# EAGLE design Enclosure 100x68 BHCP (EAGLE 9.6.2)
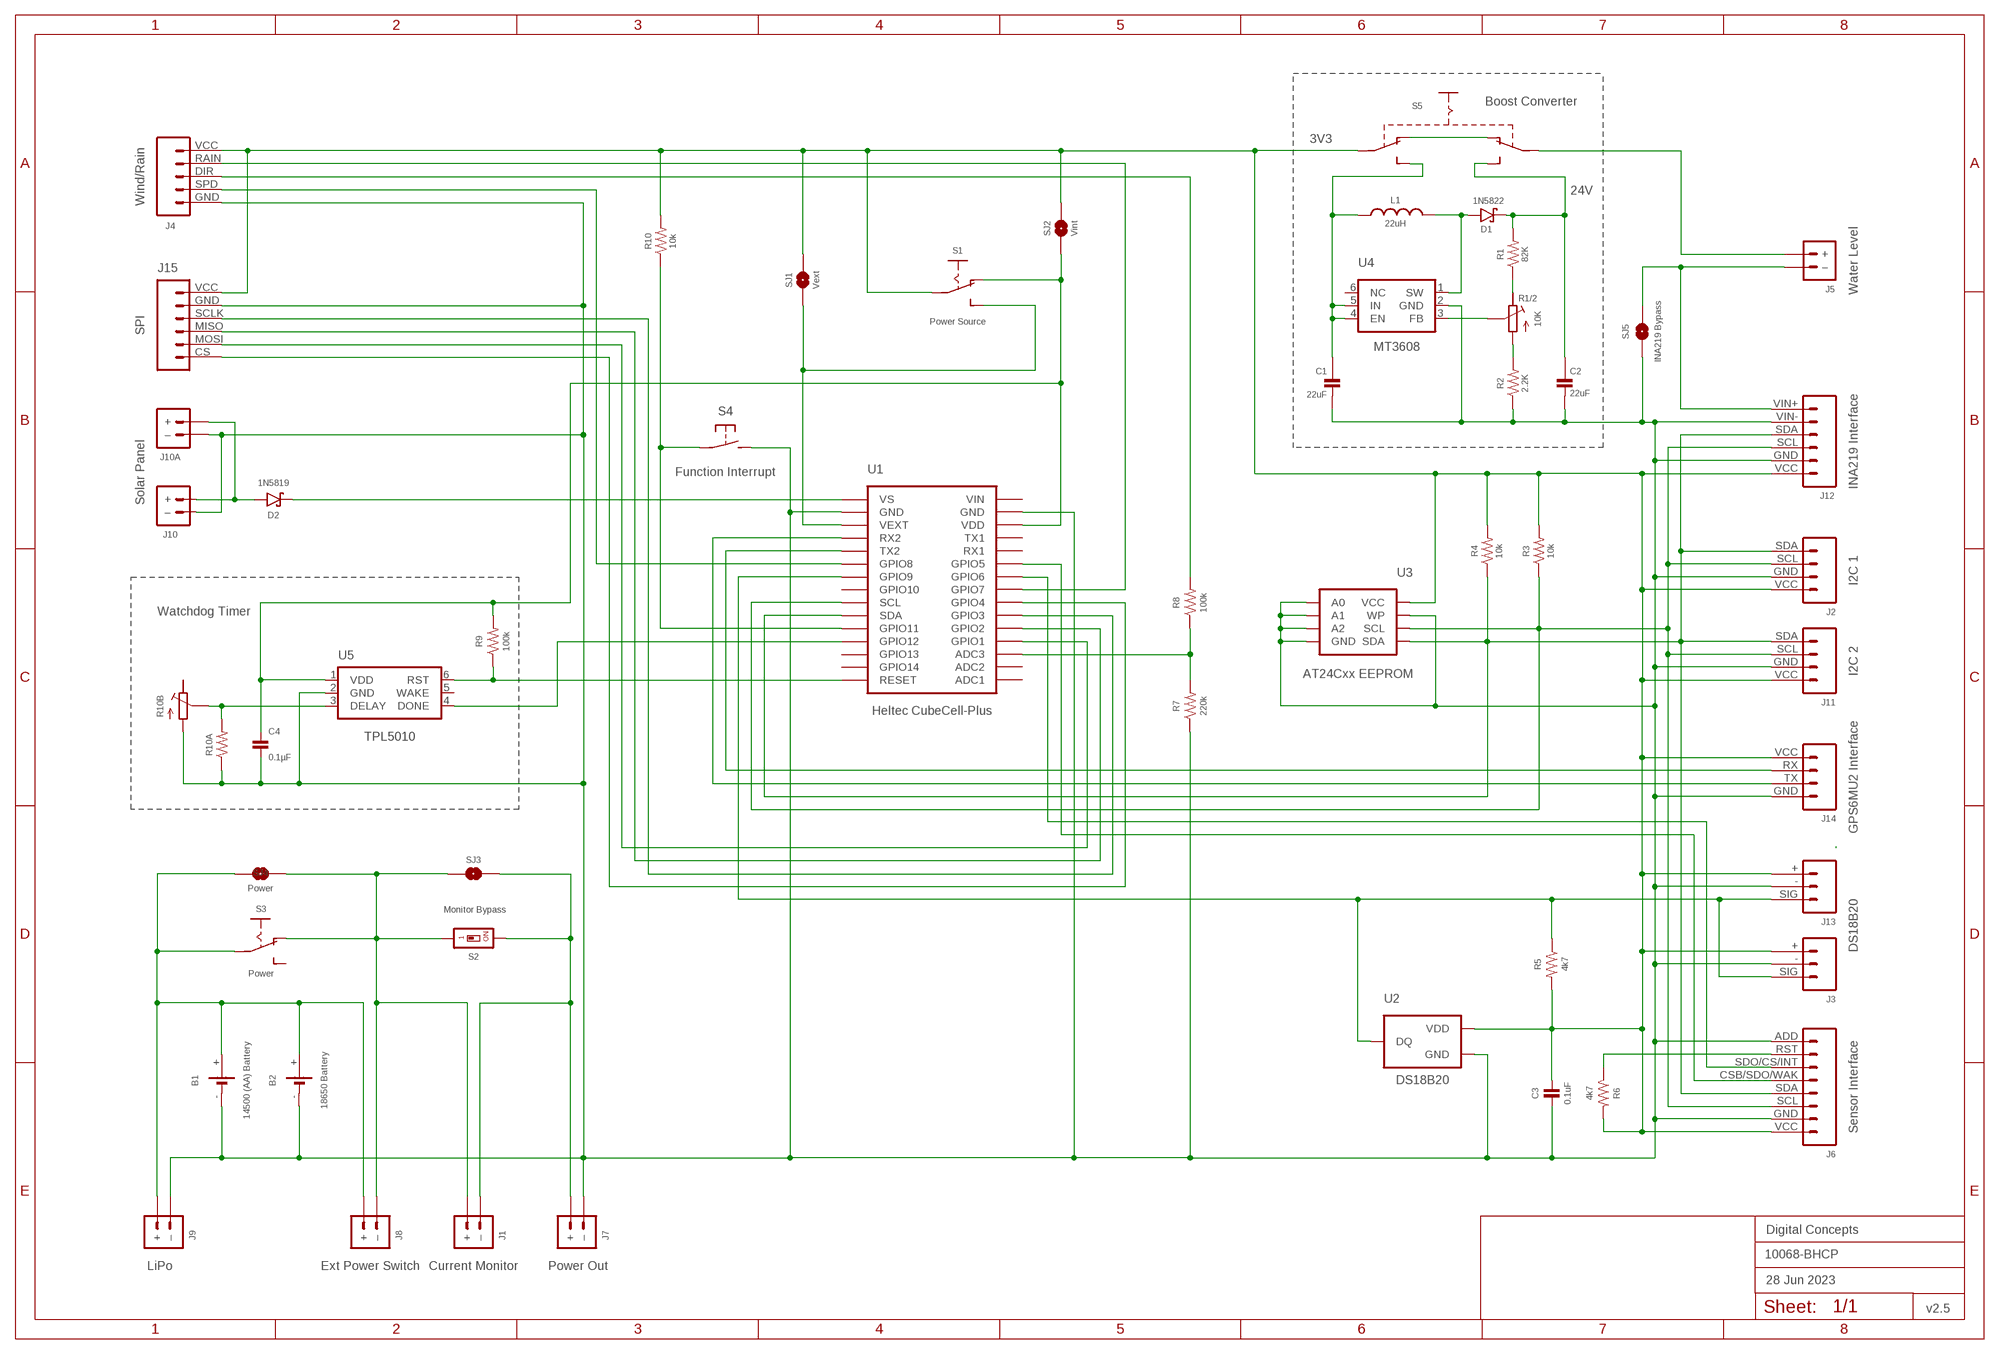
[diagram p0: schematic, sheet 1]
FRAME2 (A3L-LOC): DATE: 28 Jun 2023; OWNER: Digital Concepts; TITLE: 10068-BHCP; VERSION: v2.5

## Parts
B1  14500 (AA) Battery  BATTERY-HOLDER-14500(AA)  [BATTERY-14500]
B2  18650 Battery  BATTERY-HOLDER-18650  [BATTERY-18650]
C1  22uF  CAPACITOR-1206  [C1206]
C2  22uF  CAPACITOR-1206  [C1206]
C3  0.1uF  CAPACITOR-0805  [C0805]
C4  0.1µF  CAPACITOR-0805  [C0805]
D1  1N5822  DIODE-SCHOTTKY-1N5822  [DIODE_SMB]
D2  1N5819  1N5819-SOD-123  [SOD-123]
J1  Current Monitor  JST-PH2.0-2-HORIZONTALJST-PTH-2  [JST-PH2.0-2-HORIZONTAL]
J2  I2C 1  JST-PH2.0-4-VERTICAL-I2C  [JST-PH2.0-4-VERTICAL-I2C]
J3  DS18B20  JST-PH2.0-3-VERTICAL-DS18B20  [JST-PH2.0-3-VERTICAL-SIG]
J4  Wind/Rain  JST-PH2.0-5-DUAL-WEATHER  [JST-PH2.0-5-DUAL-WEATHER]
J5  Water Level  JST-PH2.0-2-DUAL-POWERJST-PTH-2  [JST-PH2.0-2-DUAL-POWER]
J6  Sensor Interface  HEADER-1X8-SENSOR  [CONN_08-SENSOR]
J7  Power Out  JST-GH1.25-2-HORIZONTAL-POWER  [JST-GH1.25-2-HORIZONTAL]
J8  Ext Power Switch  JST-PH2.0-2-DUAL-POWERJST-PTH-2  [JST-PH2.0-2-DUAL-POWER]
J9  LiPo  JST-PH2.0-2-HORIZONTAL-POWERJST-PTH-2  [JST-PH2.0-2-HORIZONTAL-POWER]
J10  Solar Panel  JST-PH2.0-2-VERTICAL  [JST-PH2.0-2-VERTICAL=POWER]
J10A  JST-PH2.0-2-HORIZONTAL-POWERJST-PTH-2  [JST-PH2.0-2-HORIZONTAL-POWER]
J11  I2C 2  JST-PH2.0-I2C-MALE-HORIZONTAL  [JST-PH2.0-4-HORIZONTAL]
J12  INA219 Interface  INA219-I2C-MODULE  [CONN_06-INA219]
J13  JST-PH2.0-3-HORIZONTAL-DS18B20  [JST-PH2.0-DS18B20-HORIZONTAL]
J14  GPS6MU2 Interface  HEADER-1X4-GPS  [CONN_04-GPS]
J15  SPI  JST-PH2.0-6-HORIZONTAL-SPI  [JST-PH2.0-6-HORIZONTAL-SPI]
L1  22uH  INDUCTOR-CDRH104R/6D28L5038P  [CDRH104R+6D28]
R1  82K  RESISTORR0805  [R0805]
R1/2  10K  RESISTOR-TRIMM-BAOTER-HORIZONTAL  [RTRIM64P]
R2  2.2K  RESISTORR0805  [R0805]
R3  10k  RESISTORR0805  [R0805]
R4  10k  RESISTORR0805  [R0805]
R5  4k7  RESISTORR0805  [R0805]
R6  4k7  RESISTORR0805  [R0805]
R7  220k  RESISTORR0805  [R0805]
R8  100k  RESISTORR0805  [R0805]
R9  100k  RESISTORR0805  [R0805]
R10  10k  RESISTORR0805  [R0805]
R10A  RESISTORR0805  [R0805]
R10B  RESISTOR-TRIMM-33  [RTRIM3*3]
S1  Power Source  SWITCH-SLIDE-SPDT-SMT  [SWITCH-SPDT-SMT]
S2  Monitor Bypass  SWITCH-DIP-SWS001  [SMD-001]
S3  Power  SWITCH-SLIDE-SPDT-PTH  [SWITCH-SPDT-PTH]
S4  Function Interrupt  SWITCH-MOMENTARY-2-PIN  [SWITCH-2-PAD]
S5  SWITCH-SLIDE-DPDT-PTH-S  [SWITCH-DPDT-PTH]
SJ1  Vext  SJ  [SJ]
SJ2  Vint  SJ-V-12  [SJ-VIA-12]
SJ3  Monitor  SJ  [SJ]
SJ4  Power  SJ  [SJ]
SJ5  INA219 Bypass  SJ  [SJ]
U1  Heltec CubeCell-Plus  HELTEC-CUBECELL-PLUS-X  [HELTEC-CUBECELL=PLUS-X]
U2  DS18B20  THERMOMETER-DS18B20  [TO-92]
U3  AT24Cxx EEPROM  AT24CXX-EEPROM  [SOP-8]
U4  MT3608  [SOT-23-6]
U5  TPL5010  TPL5010DDCR  [SOT-23-6]

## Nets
GND: B1.- B2.- C1.2 C2.2 C3.2 C4.2 J2.GND J3.- J4.GND J6.ADD J6.GND J7.-(–) J9.-(–) J10.-(–) J10A.-(–) J11.GND J12.GND J12.VIN- J13.- J14.GND J15.GND R2.1 R7.1 R10A.1 R10B.1(A) S4.P$2(S) SJ5.1 U1.GND@14(GND) U1.GND@17(GND) U2.1(GND) U3.P$1(A0) U3.P$2(A1) U3.P$3(A2) U3.P$4(GND) U3.P$7(WP) U4.2(GND) U5.2(GND)
N$1: D2.A J10.+ J10A.+
N$2: R7.2 R8.1 U1.ADC3
N$3: J1.2(–) J7.+ S2.2 SJ3.1
N$4: B1.+ B2.+ J8.+ J9.+ S3.2(P) SJ4.2
N$5: D2.C U1.VS
N$6: D1.A L1.1 U4.1(SW)
N$7: J4.DIR R8.2
N$8: J2.SCL J6.SCL J11.SCL J12.SCL R3.1 U1.SCL U3.P$6(SCL)
N$9: J6.RST R6.1
N$10: J6.CSB/SDO/WAK U1.GPIO5
N$11: J2.SDA J6.SDA J11.SDA J12.SDA R4.1 U1.SDA U3.P$5(SDA)
N$12: J4.SPD U1.GPIO8
N$13: S1.3(S) SJ1.1 U1.VEXT
N$14: J14.RX U1.TX2
N$15: J5.-(–) J12.VIN+ SJ5.2
N$16: J14.TX U1.RX2
N$18: R10A.2 R10B.2(S) U5.3(DELAY)
N$19: J6.SDO/CS/INT U1.GPIO6
N$20: J5.+ S5.P$2(P1)
N$21: J1.1(+) J8.-(–) S2.1 S3.1(O) SJ3.2 SJ4.1
N$22: R1/2.2(S) U4.3(FB)
N$23: R1/2.1(A) R2.2
N$24: J3.SIG J13.SIG R5.1 U1.GPIO9 U2.2(DQ)
N$25: C1.1 L1.2 S5.P$6(S2) U4.4(EN) U4.5(IN)
N$26: S5.P$1(O1) S5.P$4(O2)
N$27: R10.1 S4.P$1(P) U1.GPIO11
N$28: C2.1 D1.C R1.2 S5.P$3(S1)
N$29: J15.MOSI U1.GPIO1
N$30: J15.MISO U1.GPIO2
N$32: J4.RAIN U1.GPIO7
N$34: R9.1 U1.RST(RESET) U5.6(RST)
N$35: J15.SCLK U1.GPIO3
N$36: J15.CS U1.GPIO4
N$37: U1.GPIO12 U5.4(DONE)
N$38: R1.1 R1/2.3(E)
N$39: C4.1 R9.2 S1.1(O) SJ2.1 SJ2.1@V U1.VDD U5.1(VDD)
VEXT: C3.1 J2.VCC J3.+ J4.VCC J6.VCC J11.VCC J12.VCC J13.+ J14.VCC J15.VCC R3.2 R4.2 R5.2 R6.2 R10.2 S1.2(P) S5.P$5(P2) SJ1.2 SJ2.2 SJ2.2@V U2.3(VDD) U3.P$8(VCC)
Unconnected: R10B.3(E) S3.3(S) U1.ADC1 U1.ADC2 U1.GPIO10 U1.GPIO13 U1.GPIO14 U1.RX1 U1.TX1 U4.6(NC) U5.5(WAKE)

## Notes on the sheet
- Boost Converter
- 3V3
- 24V
- Watchdog Timer

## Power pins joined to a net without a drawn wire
VIN: U1.VIN

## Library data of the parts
B1 = digitalconcepts:BATTERY-HOLDER-14500(AA): 14500 (AA) battery holder
B2 = digitalconcepts:BATTERY-HOLDER-18650: 18650 Battery Holder
C1 C2 = digitalconcepts:CAPACITOR-1206: 1206 Capacitor
C3 C4 = digitalconcepts:CAPACITOR-0805: 0805 Capacitor
D1 = digitalconcepts:DIODE-SCHOTTKY-1N5822: 1N5822 Schottky Diode SMB
D2 = digitalconcepts:1N5819-SOD-123: 1N5819 Schottky Diode SOD-123
J1 = digitalconcepts:JST-PH2.0-2-HORIZONTAL: PH2.0 2P Right Angle PCB Connector; PROD_ID: CONN-09863; SKU: PRT-09914
J2 = digitalconcepts:JST-PH2.0-4-VERTICAL-I2C: PH2.0 4P I2C Vertical Connector
J3 = digitalconcepts:JST-PH2.0-3-VERTICAL-DS18B20: DS18B20 PH2.0 Vertical PCB Connector
J4 = digitalconcepts:JST-PH2.0-5-DUAL-WEATHER: PH2.0 5P Dual Connector
J5 J8 = digitalconcepts:JST-PH2.0-2-DUAL-POWER: JST PH2.0 2P PTH Dual-Side Connector (Power); PROD_ID: CONN-09863; SKU: PRT-09914
J6 = digitalconcepts:HEADER-1X8-SENSOR: IoT Sensors 1x8 Pin Header for 'Sandwich' IoT Sensors
J7 = digitalconcepts:JST-GH1.25-2-HORIZONTAL-POWER: JST GH1.25 2P PTH Connector (Power)
J9 J10A = digitalconcepts:JST-PH2.0-2-HORIZONTAL-POWER: PH2.0 2P Right Angle PCB Connector; PROD_ID: CONN-09863; SKU: PRT-09914
J10 = digitalconcepts:JST-PH2.0-2-VERTICAL: PH2.0 2P PCB Connector
J11 = digitalconcepts:JST-PH2.0-I2C-MALE-HORIZONTAL: PH2.0 4P (I2C) Right Angle PCB Connector
J12 = digitalconcepts:INA219-I2C-MODULE: INA219 I2C Module
J13 = digitalconcepts:JST-PH2.0-3-HORIZONTAL-DS18B20: DS18B20 PH2.0 Right Angle PCB Connector
J14 = digitalconcepts:HEADER-1X4-GPS: NEO GPS 4-Pin Header
J15 = digitalconcepts:JST-PH2.0-6-HORIZONTAL-SPI: PH2.0 6P Horizontal Connector—SPI
L1 = digitalconcepts:INDUCTOR-CDRH104R/6D28: Inductor; SPICEPREFIX: L
R1-R10 R10A = digitalconcepts:RESISTOR: Resistor; SPICEPREFIX: R
R1/2 = digitalconcepts:RESISTOR-TRIMM-BAOTER-HORIZONTAL: Trimm Resistor - Horizontal BAOTER
R10B = digitalconcepts:RESISTOR-TRIMM-3*3: Trimm Resistor - 3*3 SMD
S1 = digitalconcepts:SWITCH-SLIDE-SPDT-SMT: Mini Sliding Switch SPDT SMT
S2 = digitalconcepts:SWITCH-DIP-SWS001: SMD Dip Switch 1 pol.
S3 = digitalconcepts:SWITCH-SLIDE-SPDT-PTH: Mini Sliding Switch SPDT PTH
S4 = digitalconcepts:SWITCH-MOMENTARY-2-PIN: 2 Pin Momentary Switch
S5 = digitalconcepts:SWITCH-SLIDE-DPDT-PTH-S: Switch DPDT PTH-S
SJ1 SJ3-SJ5 = digitalconcepts:SJ: Solder Jumper
SJ2 = digitalconcepts:SJ-V-12: Solder Jumper with Pad Vias
U1 = digitalconcepts:HELTEC-CUBECELL-PLUS-X: Heltec CubeCell Dev-Board Plus Excluding internal pins
U2 = digitalconcepts:THERMOMETER-DS18B20: Digital Thermometer -55C-125C TO92-3; AVAILABILITY: Bad; DESCRIPTION: Temperature Sensor Digital, Local -55°C ~ 125°C 12 b 8-uMAX; MF: Maxim Integrated; MP: DS18B20; PACKAGE: TO-92 Maxim Integrated; PRICE: None
U3 = digitalconcepts:AT24CXX-EEPROM: AT24Cxx EEPROM SOP-8
U4 = digitalconcepts:MT3608: MT3608 DC-DC Step-Up Voltage Converter
U5 = digitalconcepts:TPL5010DDCR: TPL5010 Nano-Power System Timer with Watchdog

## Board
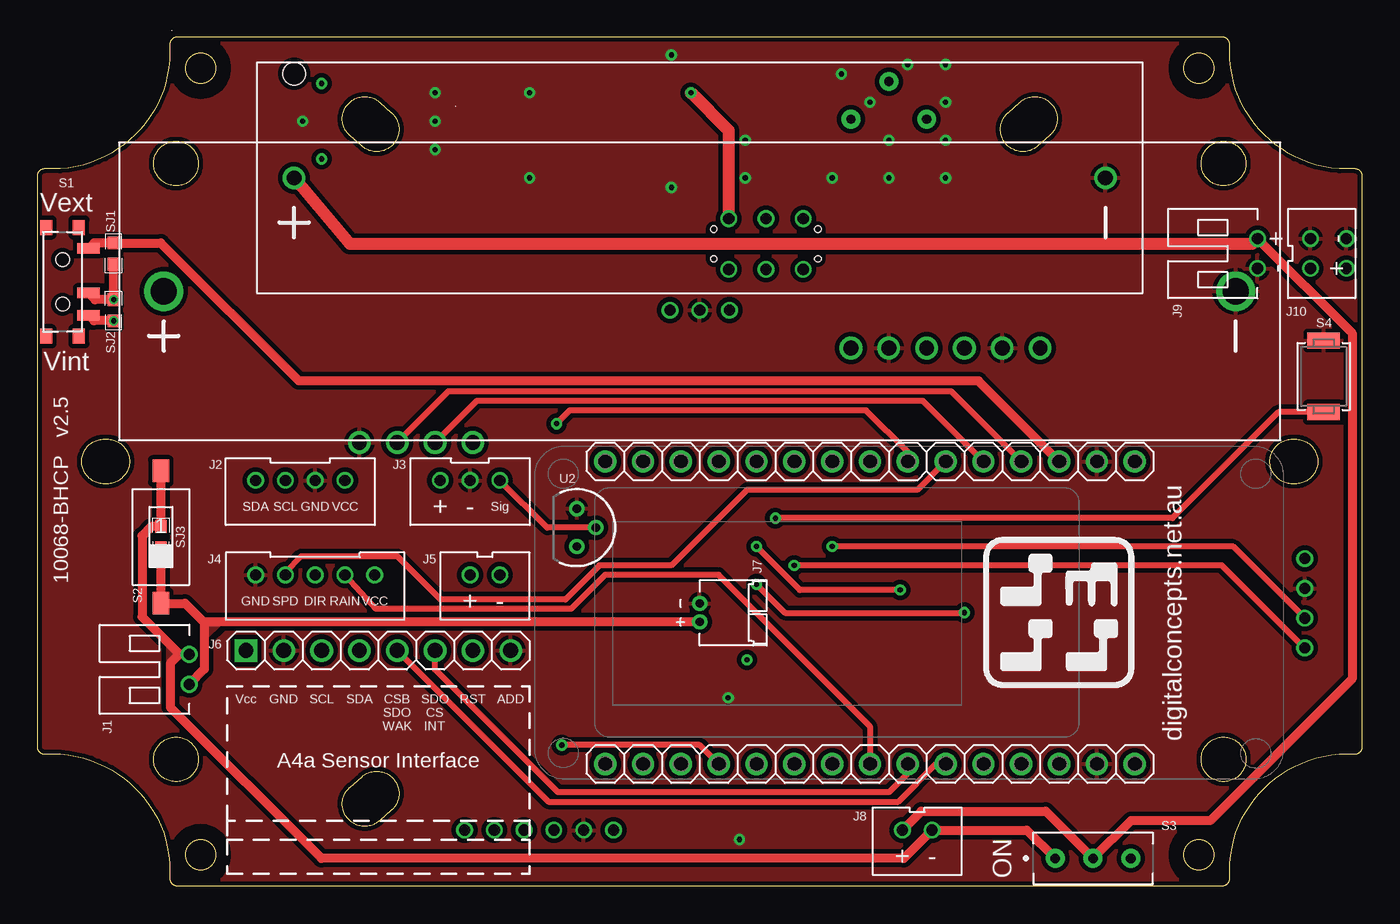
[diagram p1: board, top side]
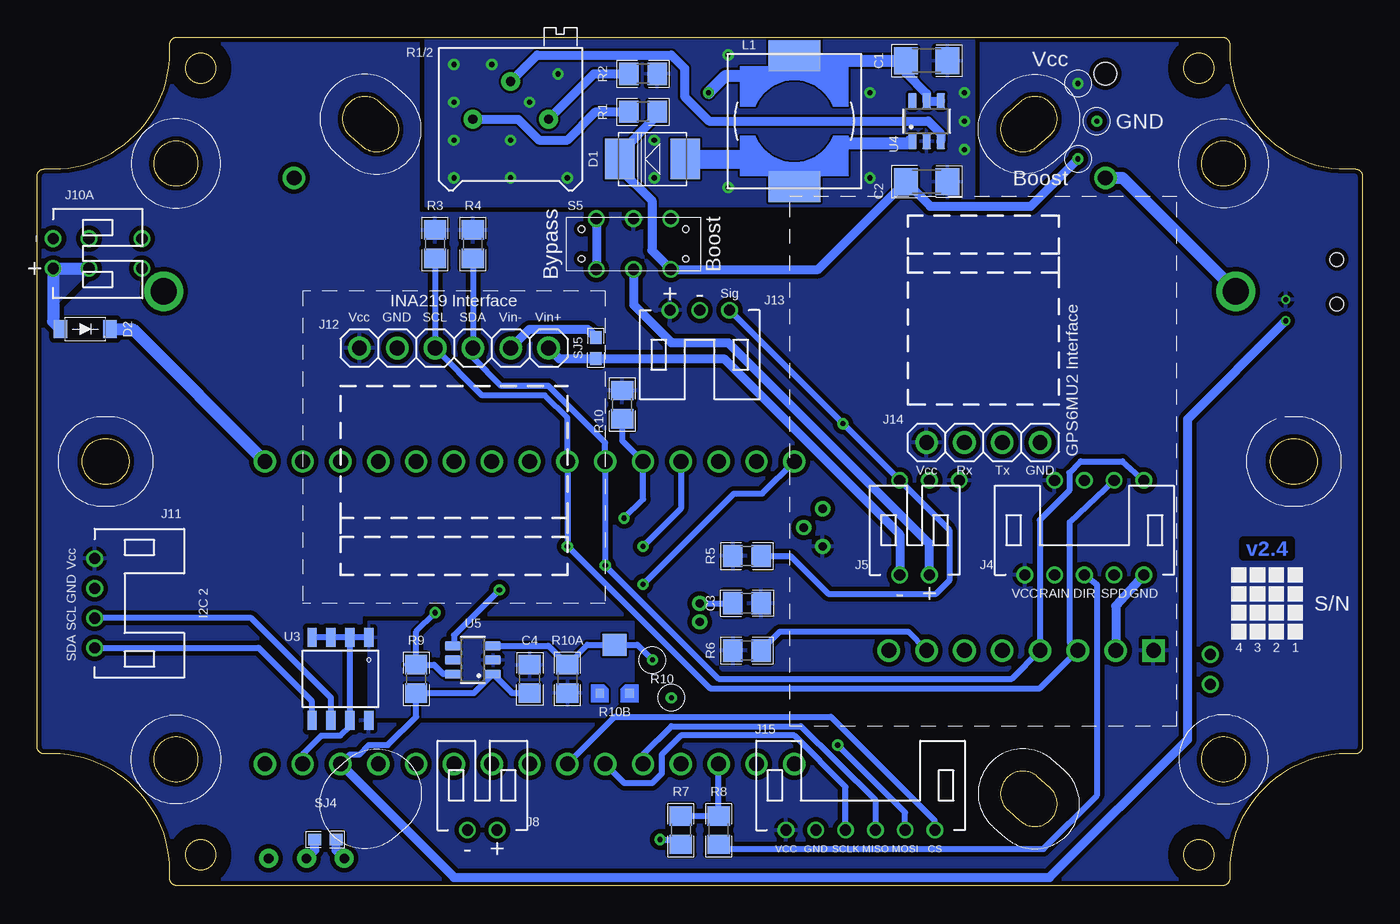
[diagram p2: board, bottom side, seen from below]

Size 89 x 57 mm. Coordinates in mm from the lower left corner, seen from the top.
Outline: 1134 segments
Outline: circle at 10.97,2.08 radius 1.02
Outline: circle at 10.97,54.92 radius 1.02
Outline: circle at 78.03,54.92 radius 1.02
Outline: circle at 78.03,2.08 radius 1.02
Copper layers (1*16): Top 0.035mm / dielectric 1.5mm / Bottom 0.035mm
Design rules "default *": minimum track width 6mil, minimum drill 0.35mm, track to track 6mil, track to pad 6mil, pad to pad 6mil, via to via 6mil, smd to smd 6mil, copper to edge 6mil, drill to drill 6mil, minimum pad ring 1mil, minimum via ring 8mil, stop-mask expansion 4mil, vias tented up to drill 0mil, thermal gap 10mil

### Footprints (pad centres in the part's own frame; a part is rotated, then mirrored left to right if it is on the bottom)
BATTERY-14500 = drill 1: + -27.25,0; - 27.25,0 | hole 1.524: -27.25,7
BATTERY-18650 = drill 1.75: + -36,0; - 36,0
C1206 = smd 1.6 x 1.8: 1 -1.4,0; 2 1.4,0
C0805 = smd 1.3 x 1.5: 1 -0.95,0; 2 0.95,0
DIODE_SMB = smd 2 x 2.7: A 2.2,0; C -2.2,0
SOD-123 = smd 0.91 x 1.22: A -1.65,0; C 1.65,0
JST-PH2.0-2-HORIZONTAL = drill 0.75: 1 1,0; 2 -1,0
JST-PH2.0-4-VERTICAL-I2C = drill 0.75: GND 1,0; SCL -1,0; SDA -3,0; VCC 3,0
JST-PH2.0-3-VERTICAL-SIG = drill 0.75: + -2,0; - 0,0; SIG 2,0
JST-PH2.0-5-DUAL-WEATHER = drill 0.75: DIR 0,0; GND 4,0; RAIN -2,0; SPD 2,0; VCC -4,0
JST-PH2.0-2-DUAL-POWER = drill 0.75: + 1,0; - -1,0
CONN_08-SENSOR = drill 1 pad 1.524: ADD 17.78,0; CSB/SDO/WAK 10.16,0; GND 2.54,0; RST 15.24,0; SCL 5.08,0; SDA 7.62,0; SDO/CS/INT 12.7,0 | drill 1 pad 1.524 square: VCC 0,0
JST-GH1.25-2-HORIZONTAL = drill 0.55 pad 1.016: + -0.625,0; - 0.625,0
JST-PH2.0-2-HORIZONTAL-POWER = drill 0.75: + 1,0; - -1,0
JST-PH2.0-2-VERTICAL=POWER = drill 0.75: + -1,0; - 1,0
JST-PH2.0-4-HORIZONTAL = drill 0.75: GND -1,0; SCL 1,0; SDA 3,0; VCC -3,0
CONN_06-INA219 = drill 1 pad 1.524: GND 2.54,0; SCL 5.08,0; SDA 7.62,0; VCC 0,0; VIN+ 12.7,0; VIN- 10.16,0
JST-PH2.0-DS18B20-HORIZONTAL = drill 0.75: + 2,0; - 0,0; SIG -2,0
CONN_04-GPS = drill 1 pad 1.524: GND 0,0; RX 5.08,0; TX 2.54,0; VCC 7.62,0
JST-PH2.0-6-HORIZONTAL-SPI = drill 0.75: CS 5,0; GND -3,0; MISO 1,0; MOSI 3,0; SCLK -1,0; VCC -5,0
CDRH104R+6D28 = smd 2.1 x 3.5: 1 -4.4,0; 2 4.4,0
R0805 = smd 1.3 x 1.5: 1 -0.95,0; 2 0.95,0
RTRIM64P = drill 0.61 pad 1.27: 1 0,-2.54; 2 2.54,0; 3 0,2.54
RTRIM3*3 = smd 0.6 x 0.6: 1 -1,-1.6; 3 1,-1.6 | smd 1.6 x 1.5: 2 0,1.65
SWITCH-SPDT-SMT = smd 0.7 x 1.5: 1 2.25,1.75; 2 0.75,1.75; 3 -2.25,1.75 | smd 1 x 0.8: GND@1 3.65,-1.1; GND@2 3.65,1.1; GND@3 -3.65,1.1; GND@4 -3.65,-1.1 | hole 0.9: -1.5,0; 1.5,0
SMD-001 = smd 1.1 x 1.5: 1 0,-4.45; 2 0,4.45
SWITCH-SPDT-PTH = drill 0.65 pad 1.27: 1 -2.54,0; 2 0,0; 3 2.54,0
SWITCH-2-PAD = smd 1.067 x 2.184: P$1 -2.4,0; P$2 2.4,0
SWITCH-DPDT-PTH = drill 0.75: P$1 -1.7,2.5; P$2 -1.7,0; P$3 -1.7,-2.5; P$4 1.7,2.5; P$5 1.7,0; P$6 1.7,-2.5 | hole 0.42: 1,3.5; -1,3.5; 1,-3.5; -1,-3.5
SJ = smd 0.864 x 0.762: 1 -0.711,0; 2 0.711,0
SJ-VIA-12 = smd 0.864 x 0.762: 1 -0.711,0; 2 0.711,0 | drill 0.35 pad 0.61: 1@V -0.711,0; 2@V 0.711,0
HELTEC-CUBECELL=PLUS-X = drill 1: ADC1 0,0; ADC2 0,2.54; ADC3 0,5.08; GND@14 0,33.02; GND@17 -20.32,33.02; GPIO1 0,7.62; GPIO2 0,10.16; GPIO3 0,12.7; GPIO4 0,15.24; GPIO5 0,22.86; GPIO6 0,20.32; GPIO7 0,17.78; GPIO8 -20.32,22.86; GPIO9 -20.32,20.32; GPIO10 -20.32,17.78; GPIO11 -20.32,10.16; GPIO12 -20.32,7.62; GPIO13 -20.32,5.08; GPIO14 -20.32,2.54; RST -20.32,0; RX1 0,25.4; RX2 -20.32,27.94; SCL -20.32,15.24; SDA -20.32,12.7; TX1 0,27.94; TX2 -20.32,25.4; VDD 0,30.48; VEXT -20.32,30.48; VIN 0,35.56; VS -20.32,35.56
TO-92 = drill 0.55 pad 1.016: 1 -1.27,0; 2 0,1.27; 3 1.27,0
SOP-8 = smd 0.635 x 1.27: P$1 -1.905,-2.794; P$2 -0.635,-2.794; P$3 0.635,-2.794; P$4 1.905,-2.794; P$5 1.905,2.794; P$6 0.635,2.794; P$7 -0.635,2.794; P$8 -1.905,2.794
SOT-23-6 = smd 1.1 x 0.6: 1 -1.35,0.95; 2 -1.35,0; 3 -1.35,-0.95; 4 1.35,-0.95; 5 1.35,0; 6 1.35,0.95

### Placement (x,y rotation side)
B1  44.5,47.55 0 top
B2  44.5,39.93 0 top
C1  29.26,55.42 0 bottom
C2  29.26,47.3 0 bottom
C3  41.32,18.97 180 bottom
C4  55.93,13.89 90 bottom
D1  47.67,48.82 0 bottom
D2  85.77,37.39 0 bottom
J1  10.21,14.53 90 top
J2  17.67,27.23 0 top
J3  29.07,27.23 0 top
J4  18.67,20.88 0 bottom
J5  30.07,20.88 0 bottom
J6  14.02,15.8 0 top
J7  44.5,18.34 90 top
J8  59.1,3.73 0 bottom
J9  81.96,42.47 90 top
J10  85.52,42.47 90 top
J10A  87.93,42.47 270 bottom
J11  85.14,18.97 270 bottom
J12  67.36,36.12 0 bottom
J13  44.5,38.66 180 bottom
J14  21.64,29.77 180 bottom
J15  33.7,3.73 0 bottom
L1  38.15,51.36 90 bottom
R1  48.31,51.99 0 bottom
R1/2  57.2,51.49 90 bottom
R2  48.31,54.53 180 bottom
R3  62.28,43.1 90 bottom
R4  59.74,43.1 90 bottom
R5  41.32,22.15 180 bottom
R6  41.32,15.8 180 bottom
R7  45.77,3.73 90 bottom
R8  43.23,3.73 270 bottom
R9  63.55,13.89 270 bottom
R10  49.71,32.31 90 bottom
R10A  53.39,13.89 90 bottom
R10B  50.21,14.53 0 bottom
S1  1.7,40.56 270 top
S2  8.3,23.42 180 top
S3  70.92,1.83 0 top
S4  86.41,34.21 90 top
S5  48.94,43.1 90 bottom
SJ1  5.13,42.47 270 top
SJ2  5.13,38.66 90 top
SJ3  8.3,23.42 90 top
SJ4  69.65,3.1 180 bottom
SJ5  51.48,36.12 270 bottom
U1  38.15,8.18 270 top
U2  36.24,24.05 270 top
U3  68.63,13.89 180 bottom
U4  29.26,51.36 90 bottom
U5  59.74,15.16 180 bottom

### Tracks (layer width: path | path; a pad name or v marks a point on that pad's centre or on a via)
$X
  cutout Bottom: 10.97,56.95 arc180 10.97,52.88 arc180
$X1
  cutout Bottom: 78.03,56.95 arc180 78.03,52.88 arc180
$X2
  cutout Top: 78.03,4.12 arc180 78.03,0.05 arc180
$X3
  cutout Top: 10.97,4.12 arc180 10.97,0.05 arc180
$X4
  cutout Top: 10.97,56.95 arc180 10.97,52.88 arc180
$X5
  cutout Top: 78.03,56.95 arc180 78.03,52.88 arc180
$X6
  cutout Bottom: 78.03,4.12 arc180 78.03,0.05 arc180
$X7
  cutout Bottom: 10.97,4.12 arc180 10.97,0.05 arc180
GND  (via drill 0.35)
  Bottom 0.406: v47.17,3.1 46.08,3.1 R7.1 | J7.- C3.2 | U3.P$2 U3.P$7 67.99,10.72 68.63,10.08 69.9,10.08 71.17,8.81 U1.GND@14 | U3.P$1 U3.P$2 | U3.P$2 U3.P$3 U3.P$4 | R10B.1 50.86,12.93
  Bottom 0.61: J4.GND 16.56,18.78 J6.GND | J12.VIN- 55.93,37.39 52.04,37.39 SJ5.1
  other vias: 26.72,53.26 58.47,55.17 54.02,54.53 47.55,50.09 47.55,47.55 53.39,47.55 57.2,47.55 57.2,50.09 61.01,47.55 61.01,50.09 61.01,55.17 26.72,51.36 55.93,52.63 61.01,52.63 42.59,46.91 42.59,55.8 33.07,53.26 33.07,47.55 26.72,49.45 17.83,51.36 46.4,12.62
  pour Top (isolate 0.305, rank 2): -1.65,58.87 -1.65,-1.92 90.59,-1.92 90.59,58.87
  pour Bottom: 26.08,57.07 26.08,45.64 62.91,45.64 62.91,57.07
  pour Bottom: 66.72,11.35 50.85,11.35 48.94,13.26 48.94,17.7 66.72,17.7
N$1
  Bottom 0.813: D2.A 87.93,37.9 J10A.+ J10.+
  pour Bottom (no thermals): 85.77,41.47 87.93,41.47 87.93,39.31
N$2
  Bottom 0.406: R7.2 R8.1 U1.ADC3
N$3
  Top 0.61: SJ3.1 S2.2 9.93,18.97 11.23,17.67 | 11.23,17.67 11.23,14.55 J1.2 | 11.23,17.67 11.27,17.71 J7.+
  pour Top: 11.23,17.71 11.23,16.43 12.51,17.71
N$4
  Top 0.61: J9.+ 88.31,37.12 88.31,13.89 78.79,4.37 73.46,4.37 S3.2 67.74,5 59.37,5 J8.+
  Top 0.813: J9.+ 81.6,43.1 21,43.1 B1.+
  Bottom 0.61: S3.2 70.36,2.39 SJ4.2
  Bottom 0.813: B1.+ 16.12,47.55 B2.+
N$5
  Bottom 0.813: D2.C 82.6,37.39 U1.VS
N$6
  Bottom 0.152: U4.1 30.4,50.01
  Bottom 0.406: 40.5,48.82 38.64,46.96 L1.1 37.96,46.96 35.04,49.88
  Bottom 0.813: 35.04,49.88 30.53,49.88 30.4,50.01
  Bottom 1.27: D1.A 40.5,48.82
N$7
  Bottom 0.406: J4.DIR 17.83,20.24 17.83,6.05 21.42,2.46 42.91,2.46 R8.2
N$8  (via drill 0.35)
  Top 0.406: J11.SCL 80.33,22.78 v53.39,22.78
  Bottom 0.406: J2.SCL 19.66,24.41 19.66,16.36 J6.SCL 21.64,13.26 43.82,13.26 53.35,22.78 v53.39,22.78 U1.SCL 53.39,31.42 54.91,32.94 59.1,32.94 J12.SCL R3.1 | U3.P$6 69.26,12.62 74.61,17.97 J11.SCL
N$9
  Bottom 0.406: R6.1 39.1,17.07 30.53,17.07 J6.RST
N$10
  Top 0.406: J6.CSB/SDO/WAK 34.34,5.64 57.83,5.64 60.37,8.18 U1.GPIO5
N$11  (via drill 0.35)
  Top 0.406: J11.SDA 85.12,15.97 79.56,21.51 v50.85,21.51
  Bottom 0.406: J2.SDA 16.1,28.5 18.92,28.5 19.68,27.73 19.68,26.54 21.66,24.56 21.66,15.82 J6.SDA 23.54,13.89 43.23,13.89 v50.85,21.51 U1.SDA 50.85,29.77 54.66,33.58 57.83,33.58 59.74,35.48 J12.SDA R4.1 | J11.SDA 74.14,15.97 70.53,12.37 U3.P$5
N$12
  Top 0.406: U1.GPIO8 59.1,26.59 47.67,26.59 42.59,21.51 37.77,21.51 35.48,19.23 27.1,19.23 24.18,22.15 17.73,22.15 16.67,21.08 J4.SPD
N$13
  Top 0.61: U1.VEXT 63.22,33.91 17.58,33.91 8.3,43.18 SJ1.1 3.82,43.18 S1.3
N$14
  Top 0.406: J14.RX 29.51,32.56 59.49,32.56 U1.TX2
N$15
  Bottom 0.61: J5.- 31.07,23.59 42.88,35.41 SJ5.2 53.95,35.41 J12.VIN+
N$16
  Top 0.406: J14.TX 27.61,33.2 61.39,33.2 U1.RX2
N$18  (via drill 0.35)
  Bottom 0.406: U5.3 54.66,16.11 R10A.2 52.05,16.18 R10B.2 48.69,16.18 v47.67,15.16
N$19
  Top 0.406: J6.SDO/CS/INT 26.72,14.53 34.97,6.27 57.2,6.27 58.47,7.54 U1.GPIO6
N$20
  Bottom 0.61: S5.P$2 48.94,39.02 46.4,36.48 42.59,36.48 29.07,22.96 J5.+
N$21
  Top 0.61: S2.1 SJ3.2 7.67,24.13 7.03,23.5 7.03,18.07 9.57,15.53 J1.1 9.55,15.53 8.94,14.92 8.94,11.99 19.1,1.83 58.2,1.83 J8.- 66.47,3.73 S3.1
  Bottom 0.61: S3.1 68.93,2.39 SJ4.1
  pour Top: 9.55,15.55 8.94,16.16 8.94,14.94
N$22
  Bottom 0.61: U4.3 28.31,50.51 29.16,51.36 43.86,51.36 45.52,53.01 45.52,54.92 46.4,55.8 55.42,55.8 R1/2.2
N$23
  Bottom 0.61: R1/2.1 51.61,54.53 R2.2
N$24  (via drill 0.35)
  Top 0.406: U1.GPIO9 58.47,29.13 55.68,31.93 35.77,31.93 v34.88,31.04 | U2.2 34.24,24.05 J3.SIG
  Bottom 0.406: R5.1 38.4,22.15 35.86,19.61 28.62,19.61 27.74,20.5 27.74,23.9 J3.SIG v34.88,31.04 J13.SIG
N$25  (via drill 0.35)
  Top 0.813: v43.9,53.26 46.44,50.72 S5.P$6
  Bottom 0.61: C1.1 30.66,54.61 29.26,53.21 U4.5 U4.4
  Bottom 0.813: C1.1 37.68,55.42 L1.2 38.53,55.76 39.88,54.41 42.76,54.41 v43.9,53.26
N$26
  Bottom 0.61: S5.P$4 S5.P$1
N$27  (via drill 0.35)
  Top 0.406: S4.P$1 83.37,31.81 76.25,24.69 v49.58,24.69
  Bottom 0.406: v49.58,24.69 48.31,25.96 U1.GPIO11 49.71,29.9 R10.1
N$28  (via drill 0.35)
  Bottom 0.61: v19.1,48.82 22.27,45.64 29.01,45.64 C2.1 36.55,41.4 S5.P$3 47.71,42.67 47.71,46.02 49.87,48.18 D1.C 50,48.95 50,49.07 47.36,51.71 R1.2
N$29  (via drill 0.35)
  Top 0.406: U1.GPIO1 44.5,9.45 v35.23,9.45
  Bottom 0.406: v35.23,9.45 30.7,4.92 J15.MOSI
N$30
  Bottom 0.406: J15.MISO 32.7,5.76 37.71,10.72 46.4,10.72 48.31,8.81 U1.GPIO2
N$32
  Top 0.406: J4.RAIN 22.75,18.59 35.86,18.59 38.15,20.88 45.77,20.88 55.93,10.72 U1.GPIO7
N$34  (via drill 0.35)
  Top 0.406: v48.31,20.24 50.21,18.34 v62.28,18.34
  Bottom 0.406: U5.6 61.72,14.21 62.36,14.85 64.18,14.85 64.17,14.84 R9.1 63.55,17.07 v62.28,18.34 | U1.RST 40.31,26.34 42.21,26.34 v48.31,20.24
N$35
  Bottom 0.406: J15.SCLK 34.7,6.64 38.15,10.08 45.77,10.08 47.04,8.81 47.04,7.54 47.67,6.91 49.58,6.91 U1.GPIO3
N$36
  Bottom 0.406: J15.CS 28.7,4.37 35.69,11.35 50.21,11.35 U1.GPIO4
N$37  (via drill 0.35)
  Top 0.406: v48.31,22.78 51.23,19.86 v57.96,19.86
  Bottom 0.406: U5.4 61.01,16.19 61.01,16.82 v57.96,19.86 | U1.GPIO12 45.77,25.32 v48.31,22.78
N$38
  Bottom 0.61: R1/2.3 56.69,51.49 55.29,50.09 53.39,50.09 51.48,51.99 R1.1
N$39
  Top 0.61: SJ2.1@V 3.82,37.95 S1.1
  Bottom 0.406: C4.1 57.12,12.94 U5.1 59.66,12.94 R9.2 63.55,11.35 65.45,9.45 66.72,9.45 67.36,8.81 67.99,8.81 U1.VDD
  Bottom 0.61: U1.VDD 61.01,0.56 21,0.56 11.73,9.83 11.73,31.34 SJ2.1@V
VEXT  (via drill 0.35)
  Top 0.61: S1.2 3.89,39.37 SJ2.2@V SJ1.2
  other vias: 19.1,53.9
  pour Bottom (isolate 0.305, rank 2): -0.65,57.87 -0.65,-0.92 89.59,-0.92 89.59,57.87

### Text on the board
Bottom: v2.4
tPlace: 10068-BHCP v2.5 | digitalconcepts.net.au | Vcc | GND | SCL | SDA | RST | ADD | CSB / SDO / WAK | SDO / CS / INT
bPlace: Vin+ | Vin- | SDA | SCL | GND | Vcc | GND | Tx | Rx | Vcc | S/N | 1 | 2 | 3 | 4
tNames: Vext | Vint | A4a Sensor Interface | ON
bNames: Vcc | GND | Boost | Boost | Bypass | Vcc | J4 | J5 | GND | SCL | SDA | R10 | J8
tValues: INT | Water Level
bValues: Wind/Rain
